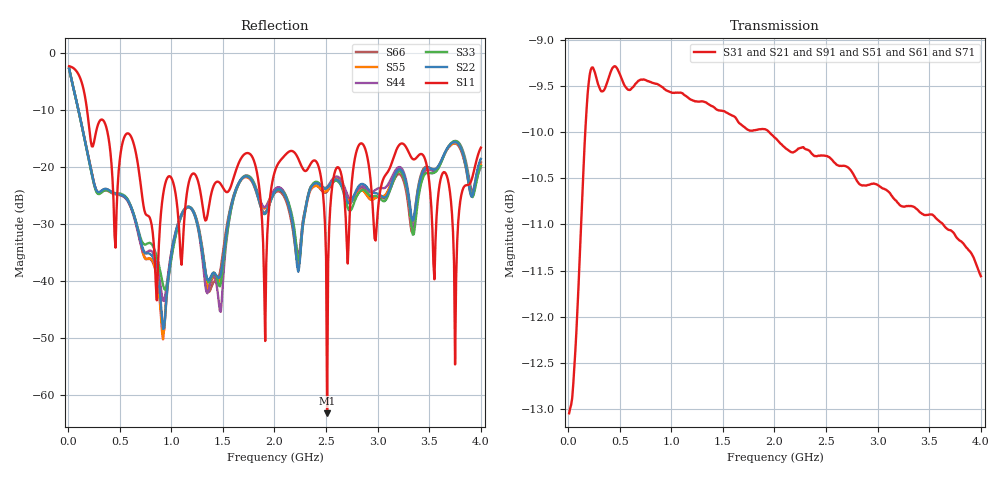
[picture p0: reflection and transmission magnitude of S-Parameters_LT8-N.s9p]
! MTS Systemtechnik GmbH
! S-Parameters
! Model: RK3-2xLT2-588P
! Rohde & Schwarz ZVB8 2Ports - Version 3.20 - 1145.1010k08 SN: 100119
! Converted & adapted with MATLAB
!		|  MTS  |
!		|  |--o OUT 8 (Port 9)
!		|  |--o OUT 7 (Port 8)
!		|  |--o OUT 6 (Port 7)
!		|  |--o OUT 5 (Port 6)
! C (Port 1) o--| LT8-588P-4G |
!		|  |--o OUT 4 (Port 5)
!		|  |--o OUT 3 (Port 4)
!		|  |--o OUT 2 (Port 3)
!		|  |--o OUT 1 (Port 2)
! S9P File: Measurements:
! <S11,S12,S13,S14,S15,S16,S17,S18,S19>,
! <S21,S22,S23,S24,S25,S26,S27,S28,S29>,
! <S31,S32,S33,S34,S35,S36,S37,S38,S39>,
! <S41,S42,S43,S44,S45,S46,S47,S48,S49>,
! <S51,S52,S53,S54,S55,S56,S57,S58,S59>,
! <S61,S62,S63,S64,S65,S66,S67,S68,S69>,
! <S71,S72,S73,S74,S75,S76,S77,S78,S79>,
! <S81,S82,S83,S84,S85,S86,S87,S88,S89>,
! <S91,S92,S93,S94,S95,S96,S97,S98,S99>:
# HZ  S  DB  R  50.00
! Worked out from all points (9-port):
!   400 points, 10 MHz to 4 GHz, reference 50 ohm
!   strongest paths, dB at 10 MHz, 1.01 GHz, 2.01 GHz, 3.01 GHz, 4 GHz:
!     S31: -13.1, -9.6, -10.1, -10.6, -11.6
!     S21: -13.0, -9.6, -10.1, -10.6, -11.6
!     S91: -13.0, -9.6, -10.1, -10.6, -11.7
!     S51: -13.0, -9.6, -10.1, -10.6, -11.6
!     S61: -13.0, -9.6, -10.1, -10.6, -11.6
!     S71: -13.0, -9.6, -10.1, -10.6, -11.6
!   lowest |S11| = -63.2 dB at 2.51 GHz (marker M1), VSWR 1.00, Z = 50 + j0.0633 ohm
!   |S11| at or under -10 dB: 184.2 MHz to end of sweep
